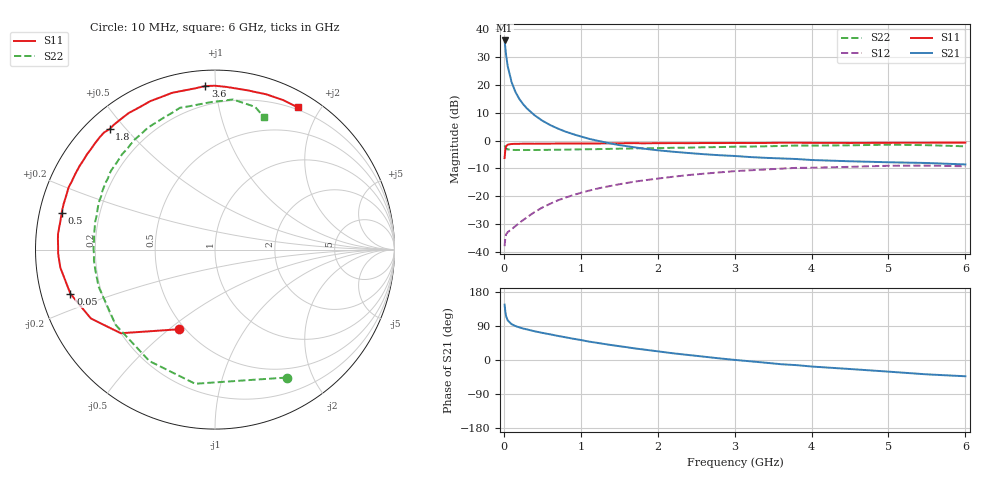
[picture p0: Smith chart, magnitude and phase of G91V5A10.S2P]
! SIEMENS Small Signal Semiconductors
! BFG235
! Si NPN RF Bipolar Junction Transistor in SOT223
! VCE = 1.5 V  IC = 100 mA
! Common Emitter S-Parameters:  July  1994
# GHz  S  MA  R  50
!  f  S11  S21  S12  S22
! GHz  MAG  ANG  MAG  ANG  MAG  ANG  MAG  ANG
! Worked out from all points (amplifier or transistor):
!   40 points, 10 MHz to 6 GHz, reference 50 ohm
!   highest |S21| = 35.9 dB at 10 MHz (marker M1)
!   |S21| within 3 dB of that: start of sweep to 20.75 MHz
!   unconditionally stable (mu >= 1): 438.9 MHz to 1.62 GHz; 1.759 GHz to 1.893 GHz
!   at 200 MHz: K = 0.79, MSG = 22.2 dB, |S12| = -29.5 dB
!   at 1.5 GHz: K = 1.01, MAG = 6.3 dB, |S12| = -15.7 dB
!   at 6 GHz: K = 0.95, MSG = 0.3 dB, |S12| = -9.2 dB
!   S11 on the Smith chart (normalised r, x): 10 MHz: 0.47, -0.54; 50 MHz: 0.09, -0.15; 500 MHz: 0.07, +0.12; 1.8 GHz: 0.07, +0.45; 3.6 GHz: 0.09, +0.94; 6 GHz: 0.17, +1.72
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0.01  0.486 -114.1  62.14 146.1  0.0128 57.1  0.8166 -60.8
0.02  0.702 -138.4  44.96 126.3  0.0184 41.0  0.7555 -98.4
0.03  0.791 -151.0  33.62 115.3  0.0209 34.8  0.7206 -120.5
0.05  0.8423 -163.0  21.57 104.7  0.0228 29.1  0.6944 -142.8
0.1  0.8674 -173.3  11.19 94.7  0.0257 33.3  0.6806 -162.4
0.15  0.8743 -178.5  7.476 89.6  0.0292 39.8  0.6764 -170.3
0.2  0.8742 179.0  5.59 86.2  0.0334 44.9  0.6775 -174.7
0.25  0.8772 176.1  4.502 83.1  0.0375 48.6  0.6747 -177.8
0.3  0.879 174.1  3.759 80.7  0.0421 51.7  0.6768 179.5
0.4  0.8758 170.0  2.833 75.8  0.0524 55.5  0.6759 175.7
0.5  0.8788 166.4  2.27 71.6  0.063 57.1  0.6791 172.5
0.6  0.8808 163.4  1.902 67.8  0.0734 57.6  0.6814 169.5
0.7  0.882 159.8  1.643 63.7  0.0845 57.7  0.6854 166.8
0.9  0.8838 154.5  1.302 56.2  0.1051 55.8  0.69 161.9
1.1  0.8868 148.2  1.08 48.8  0.1259 53.1  0.6993 157.1
1.8  0.8922 131.2  0.72 28.1  0.1916 41.1  0.7276 142.4
2.2  0.9 122.3  0.63 17.7  0.2245 33.4  0.7416 134.3
3.2  0.9031 101.2  0.506 -3.4  0.293 14.1  0.7796 115.4
3.6  0.9129 93.4  0.478 -11.1  0.3135 5.8  0.7994 107.2
4.5  0.9056 78.3  0.425 -23.8  0.3381 -9.8  0.8217 91.7
5.5  0.9154 65.5  0.396 -37.9  0.356 -27.3  0.8261 74.3
6  0.9171 59.9  0.373 -42.9  0.3456 -33.8  0.7875 69.8
